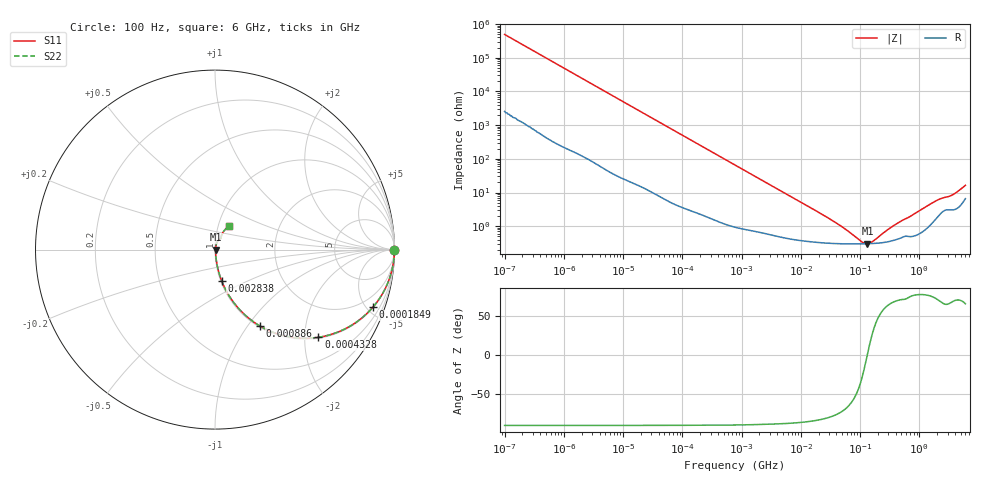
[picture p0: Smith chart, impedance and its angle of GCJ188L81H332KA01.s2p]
!Murata Part Number: GCJ188L81H332KA01
!These Parameters are Measured in Series Mode Connection
!Data Generated on Mar 13, 2026
!  o--ll--o
!Port1  Port2
!  o------o
!Operation Temp=25[degC], DC Bias Voltage=0[V]
!Freq. Start=100[Hz] Stop=6[GHz] 401[Steps]
# Hz S RI R 50
!Freq.(Hz) S11(Real) S11(Imag) S21(Real) S21(Imag) S12(Real) S12(Imag) S22(Real) S22(Imag)
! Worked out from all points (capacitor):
!   401 points, 100 Hz to 6 GHz, reference 50 ohm
!   read as one part in series: C = 3.24 nF near 109 Hz
!   lowest |Z| = 302 mohm at 133.4 MHz (marker M1)
!   series resonance near 131.9 MHz, so ESL is about 450 pH
!   S11 on the Smith chart (normalised r, x): 100 Hz: open; 184.9 kHz: 1.05, -5.44; 432.8 kHz: 1.03, -2.33; 886 kHz: 1.02, -1.14; 2.838 MHz: 1.01, -0.36; 6 GHz: 1.13, +0.30
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100  1 -0.000204  1.1e-06 0.000204  1.1e-06 0.000204  1 -0.000204
2008  1 -0.00406  3.66e-05 0.00406  3.66e-05 0.00406  1 -0.00406
12592  0.9992 -0.0253  0.000775 0.0253  0.000775 0.0253  0.9992 -0.0253
40335  0.993 -0.08  0.00695 0.08  0.00695 0.08  0.993 -0.08
98762  0.9614 -0.189  0.0386 0.189  0.0386 0.189  0.9614 -0.189
184852  0.8788 -0.322  0.1212 0.322  0.1212 0.322  0.8788 -0.322
276587  0.7664 -0.4182  0.2336 0.4182  0.2336 0.4182  0.7664 -0.4182
432798  0.5759 -0.4887  0.4241 0.4887  0.4241 0.4887  0.5759 -0.4887
774597  0.3021 -0.4521  0.6979 0.4521  0.6979 0.4521  0.3021 -0.4521
885955  0.2499 -0.4253  0.7501 0.4253  0.7501 0.4253  0.2499 -0.4253
1516199  0.1063 -0.2976  0.8937 0.2976  0.8937 0.2976  0.1063 -0.2976
2837864  0.0367 -0.1727  0.9633 0.1727  0.9633 0.1727  0.0367 -0.1727
6075234  0.0113 -0.0836  0.9887 0.0836  0.9887 0.0836  0.0113 -0.0836
1.555665e7  0.00448 -0.0329  0.9955 0.0329  0.9955 0.0329  0.00448 -0.0329
4.556224e7  0.00311 -0.0101  0.9969 0.0101  0.9969 0.0101  0.00311 -0.0101
1.066761e8  0.00298 -0.0017  0.997 0.0017  0.997 0.0017  0.00298 -0.0017
1.334425e8  0.00301 9.23e-05  0.997 -9.23e-05  0.997 -9.23e-05  0.00301 9.23e-05
1.669249e8  0.00306 0.00189  0.9969 -0.00189  0.9969 -0.00189  0.00306 0.00189
3.124326e8  0.00357 0.00772  0.9964 -0.00772  0.9964 -0.00772  0.00357 0.00772
1.791126e9  0.0168 0.0495  0.9832 -0.0495  0.9832 -0.0495  0.0168 0.0495
3.505958e9  0.0348 0.0716  0.9652 -0.0716  0.9652 -0.0716  0.0348 0.0716
6e9  0.0797 0.1289  0.9203 -0.1289  0.9203 -0.1289  0.0797 0.1289
